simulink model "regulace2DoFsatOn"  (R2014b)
settings: Solver=ode45  StartTime=0.0  StopTime=50  RelTol=1e-3
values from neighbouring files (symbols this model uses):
  p = [0.2728 0.1079 0.3077 0.0546]    [SITOrizeniP.m]    (also in SITOrizeniPD.m; normaHnekonecno.m = [1 (3*alfa(j)-a0)])
  par = [0.2728 0.1079 0.3077 0.0546 0.1370 0.0320 0.1151 0.0357]    [regulace2DoF.m]    (also in SITOrizeniP.m = [-0.0536 0.05 0.13 0.006 -0.0545 0.1 0.16 0.1746 -0.058     ; SITOrizeniPD.m = [-0.0536 0.05 0.13 0.006 -0.0545 0.1 0.16 0.1746 -0.058     ; regulace1DoF.m; regulaceMPM.m)
undefined symbols (not defined in the file or in its folder): magnitude, q, r
libraries: simulink x4

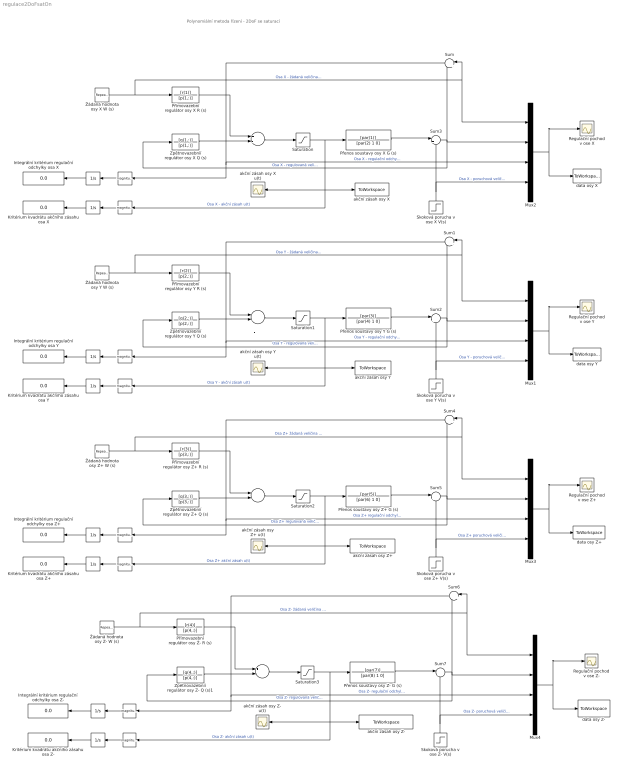
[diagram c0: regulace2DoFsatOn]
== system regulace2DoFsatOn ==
  note: Polynomiální metoda řízení - 2DoF se saturací
  " " : Math  Operator=magnitude^2
  "  " : Integrator
  "    " : Integrator
  "     " : Integrator
  "      " : Math  Operator=magnitude^2
  "       " : Math  Operator=magnitude^2
  "        " : Integrator
  "         " : Integrator
  "          " : Math  Operator=magnitude^2
  "            " : Math  Operator=magnitude^2
  "              " : Math  Operator=magnitude^2
  "               " : Integrator
  "                                " : Integrator
  "                                     " : Sum  Inputs=+-
  "                                         " : Integrator
  "                                                 " : Sum  Inputs=+-
  "                                                   " : Math  Operator=magnitude^2
  "                                                                      " : Sum  Inputs=+-
  "                                                                           " : Math  Operator=magnitude^2
  "                                                                                             " : Sum  Inputs=+-
  Integrální kritérium regulační odchylky osa X : Display
  Integrální kritérium regulační odchylky osa Y : Display
  Integrální kritérium regulační odchylky osa Z+ : Display
  Integrální kritérium regulační odchylky osa Z- : Display
  Kritérium kvadrátu akčního zásahu osa X : Display
  Kritérium kvadrátu akčního zásahu osa Y : Display
  Kritérium kvadrátu akčního zásahu osa Z+ : Display
  Kritérium kvadrátu akčního zásahu osa Z- : Display
  Mux{1..4} (4 alike) : Mux
  Přenos soustavy osy X G (s) : TransferFcn  Numerator=[par(1)]  Denominator=[par(2) 1 0]
  Přenos soustavy osy Y G (s) : TransferFcn  Numerator=[par(3)]  Denominator=[par(4) 1 0]
  Přenos soustavy osy Z+ G (s) : TransferFcn  Numerator=[par(5)]  Denominator=[par(6) 1 0]
  Přenos soustavy osy Z- G (s) : TransferFcn  Numerator=[par(7)]  Denominator=[par(8) 1 0]
  Přímovazební regulátor osy X R (s) : TransferFcn  Numerator=[r(1)]  Denominator=[p(1,:)]
  Přímovazební regulátor osy Y R (s) : TransferFcn  Numerator=[r(2)]  Denominator=[p(2,:)]
  Přímovazební regulátor osy Z+ R (s) : TransferFcn  Numerator=[r(3)]  Denominator=[p(3,:)]
  Přímovazební regulátor osy Ź- R (s) : TransferFcn  Numerator=[r(4)]  Denominator=[p(4,:)]
  Regulační pochod v ose X : Scope
  Regulační pochod v ose Y : Scope
  Regulační pochod v ose Z+ : Scope
  Regulační pochod v ose Z- : Scope
  Saturation{,1..3} (4 alike) : Saturate  UpperLimit=1  LowerLimit=-1
  Skoková porucha v ose X V(s) : Step  Time=15  After=0.1  SampleTime=0
  Skoková porucha v ose Y V(s) : Step  Time=15  After=0.1  SampleTime=0
  Skoková porucha v ose Z+ V(s) : Step  Time=15  After=0.1  SampleTime=0
  Skoková porucha v ose Z- V(s) : Step  Time=15  After=0.1  SampleTime=0
  Sum{,1,4,6} (4 alike) : Sum  Inputs=|+-
  Sum{2..3,5,7} (4 alike) : Sum  Inputs=|++
  Zpětnovazebníí regulátor osy X Q (s) : TransferFcn  Numerator=[q(1,:)]  Denominator=[p(1,:)]
  Zpětnovazebníí regulátor osy Y Q (s) : TransferFcn  Numerator=[q(2,:)]  Denominator=[p(2,:)]
  Zpětnovazebníí regulátor osy Z+ Q (s) : TransferFcn  Numerator=[q(3,:)]  Denominator=[p(3,:)]
  Zpětnovazebníí regulátor osy Z- Q (s)1 : TransferFcn  Numerator=[q(4,:)]  Denominator=[p(4,:)]
  akční zásah osy X : ToWorkspace  VariableName=akcniZasahXsat  SaveFormat=Timeseries  SampleTime=-1
  akční zásah osy X u(t) : Scope
  akční zásah osy Y : ToWorkspace  VariableName=akcniZasahYsat  SaveFormat=Timeseries  SampleTime=-1
  akční zásah osy Y u(t) : Scope
  akční zásah osy Z+ : ToWorkspace  VariableName=akcniZasahZplusSat  SaveFormat=Timeseries  SampleTime=-1
  akční zásah osy Z+ u(t) : Scope
  akční zásah osy Z- : ToWorkspace  VariableName=akcniZasahZminusSat  SaveFormat=Timeseries  SampleTime=-1
  akční zásah osy Z- u(t) : Scope
  data osy X : ToWorkspace  VariableName=dataXsat  SaveFormat=Timeseries  SampleTime=-1
  data osy Y : ToWorkspace  VariableName=dataYsat  SaveFormat=Timeseries  SampleTime=-1
  data osy Z+ : ToWorkspace  VariableName=dataZplusSat  SaveFormat=Timeseries  SampleTime=-1
  data osy Z- : ToWorkspace  VariableName=dataZminusSat  SaveFormat=Timeseries  SampleTime=-1
  Žádaná hodnota osy X W (s) : simulink/Sources/Repeating Sequence  rep_seq_t=[0 9.99 10 19.99 20 29.99 30 39.99 40 50]  rep_seq_y=[0 0 0.4 0.4 0.2 0.2 0.6 0.6 0 0]
  Žádaná hodnota osy Y W (s) : simulink/Sources/Repeating Sequence  rep_seq_t=[0 9.99 10 19.99 20 29.99 30 39.99 40 50]  rep_seq_y=[0 0 0.4 0.4 0.2 0.2 0.6 0.6 0 0]
  Žádaná hodnota osy Z+ W (s) : simulink/Sources/Repeating Sequence  rep_seq_t=[0 9.99 10 19.99 20 29.99 30 39.99 40 50]  rep_seq_y=[0 0 0.4 0.4 0.2 0.2 0.6 0.6 0 0]
  Žádaná hodnota osy Z- W (s) : simulink/Sources/Repeating Sequence  rep_seq_t=[0 9.99 10 19.99 20 29.99 30 39.99 40 50]  rep_seq_y=[0 0 0.4 0.4 0.2 0.2 0.6 0.6 0 0]
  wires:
  Žádaná hodnota osy X W (s)/1 -> Sum/1, Mux2/1, Přímovazební regulátor osy X R (s)/1  "Osa X - žádaná veličina w(t)"
  Zpětnovazebníí regulátor osy X Q (s)/1 -> "                                     "/2
  Přímovazební regulátor osy X R (s)/1 -> "                                     "/1
  "                                     "/1 -> Saturation/1
  Saturation/1 -> akční zásah osy X/1, " "/1, akční zásah osy X u(t)/1, Přenos soustavy osy X G (s)/1  "Osa X - akční zásah u(t)"
  Přenos soustavy osy X G (s)/1 -> Sum3/1
  Skoková porucha v ose X V(s)/1 -> Sum3/2, Mux2/4  "Osa X - poruchová veličina v(t)"
  Mux2/1 -> Regulační pochod v ose X/1, data osy X/1
  Sum3/1 -> Sum/2, Mux2/2, Zpětnovazebníí regulátor osy X Q (s)/1  "Osa X - regulovaná veličina y(t)"
  "     "/1 -> Kritérium kvadrátu akčního zásahu osa X/1
  " "/1 -> "     "/1
  "      "/1 -> "  "/1
  "  "/1 -> Integrální kritérium regulační odchylky osa X/1
  Sum/1 -> "      "/1, Mux2/3  "Osa X - regulační odchylka e(t)"
  Žádaná hodnota osy Y W (s)/1 -> Sum1/1, Mux1/1, Přímovazební regulátor osy Y R (s)/1  "Osa Y - žádaná veličina w(t)"
  Zpětnovazebníí regulátor osy Y Q (s)/1 -> "                                                                      "/2
  Přímovazební regulátor osy Y R (s)/1 -> "                                                                      "/1
  "                                                                      "/1 -> Saturation1/1
  Saturation1/1 -> akční zásah osy Y/1, "       "/1, akční zásah osy Y u(t)/1, Přenos soustavy osy Y G (s)/1  "Osa Y - akční zásah u(t)"
  Přenos soustavy osy Y G (s)/1 -> Sum2/1
  Skoková porucha v ose Y V(s)/1 -> Sum2/2, Mux1/4  "Osa Y - poruchová veličina v(t)"
  Mux1/1 -> Regulační pochod v ose Y/1, data osy Y/1
  Sum2/1 -> Sum1/2, Mux1/2, Zpětnovazebníí regulátor osy Y Q (s)/1  "Osa Y - regulovaná veličina y(t)"
  "        "/1 -> Kritérium kvadrátu akčního zásahu osa Y/1
  "       "/1 -> "        "/1
  "          "/1 -> "    "/1
  "    "/1 -> Integrální kritérium regulační odchylky osa Y/1
  Sum1/1 -> "          "/1, Mux1/3  "Osa Y - regulační odchylka e(t)"
  Žádaná hodnota osy Z+ W (s)/1 -> Sum4/1, Mux3/1, Přímovazební regulátor osy Z+ R (s)/1  "Osa Z+ žádaná veličina w(t)"
  Zpětnovazebníí regulátor osy Z+ Q (s)/1 -> "                                                 "/2
  Přímovazební regulátor osy Z+ R (s)/1 -> "                                                 "/1
  "                                                 "/1 -> Saturation2/1
  Saturation2/1 -> akční zásah osy Z+/1, "            "/1, akční zásah osy Z+ u(t)/1, Přenos soustavy osy Z+ G (s)/1  "Osa Z+ akční zásah u(t)"
  Přenos soustavy osy Z+ G (s)/1 -> Sum5/1
  Skoková porucha v ose Z+ V(s)/1 -> Sum5/2, Mux3/4  "Osa Z+ poruchová veličina v(t)"
  Mux3/1 -> Regulační pochod v ose Z+/1, data osy Z+/1
  Sum5/1 -> Sum4/2, Mux3/2, Zpětnovazebníí regulátor osy Z+ Q (s)/1  "Osa Z+ regulovaná veličina y(t)"
  "               "/1 -> Kritérium kvadrátu akčního zásahu osa Z+/1
  "            "/1 -> "               "/1
  "              "/1 -> "         "/1
  "         "/1 -> Integrální kritérium regulační odchylky osa Z+/1
  Sum4/1 -> "              "/1, Mux3/3  "Osa Z+ regulační odchylka e(t)"
  Žádaná hodnota osy Z- W (s)/1 -> Sum6/1, Mux4/1, Přímovazební regulátor osy Ź- R (s)/1  "Osa Z- žádaná veličina w(t)"
  Zpětnovazebníí regulátor osy Z- Q (s)1/1 -> "                                                                                             "/2
  Přímovazební regulátor osy Ź- R (s)/1 -> "                                                                                             "/1
  "                                                                                             "/1 -> Saturation3/1
  Saturation3/1 -> akční zásah osy Z- u(t)/1, akční zásah osy Z-/1, "                                                   "/1, Přenos soustavy osy Z- G (s)/1  "Osa Z- akční zásah u(t)"
  Přenos soustavy osy Z- G (s)/1 -> Sum7/1
  Skoková porucha v ose Z- V(s)/1 -> Sum7/2, Mux4/4  "Osa Z- poruchová veličina v(t)"
  Mux4/1 -> Regulační pochod v ose Z-/1, data osy Z-/1
  Sum7/1 -> Sum6/2, Mux4/2, Zpětnovazebníí regulátor osy Z- Q (s)1/1  "Osa Z- regulovaná veličina y(t)"
  "                                         "/1 -> Kritérium kvadrátu akčního zásahu osa Z-/1
  "                                                   "/1 -> "                                         "/1
  "                                                                           "/1 -> "                                "/1
  "                                "/1 -> Integrální kritérium regulační odchylky osa Z-/1
  Sum6/1 -> "                                                                           "/1, Mux4/3  "Osa Z- regulační odchylka e(t)"
